{attribute 'qualified_only'}
VAR_GLOBAL
	//FFU
	FFU1_1_STATUS	:	UINT	;	//	FFU1_1运行状态
	FFU1_2_STATUS	:	UINT	;	//	FFU1_2运行状态
	FFU1_3_STATUS	:	UINT	;	//	FFU1_3运行状态
	FFU1_4_STATUS	:	UINT	;	//	FFU1_4运行状态
	FFU1_5_STATUS	:	UINT	;	//	FFU1_5运行状态
	FFU1_6_STATUS	:	UINT	;	//	FFU1_6运行状态
	FFU2_1_STATUS	:	UINT	;	//	FFU2_1运行状态
	FFU2_2_STATUS	:	UINT	;	//	FFU2_2运行状态
	FFU2_3_STATUS	:	UINT	;	//	FFU2_3运行状态
	FFU2_4_STATUS	:	UINT	;	//	FFU2_4运行状态
	FFU2_5_STATUS	:	UINT	;	//	FFU2_5运行状态
	FFU2_6_STATUS	:	UINT	;	//	FFU2_6运行状态
	FFU3_1_STATUS	:	UINT	;	//	FFU3_1运行状态
	FFU3_2_STATUS	:	UINT	;	//	FFU3_2运行状态
	FFU3_3_STATUS	:	UINT	;	//	FFU3_3运行状态
	FFU3_4_STATUS	:	UINT	;	//	FFU3_4运行状态
	FFU3_5_STATUS	:	UINT	;	//	FFU3_5运行状态
	FFU3_6_STATUS	:	UINT	;	//	FFU3_6运行状态

	FFU1_1_SPEED_PV	:	UINT	;	//	FFU1_1当前转速
	FFU1_2_SPEED_PV	:	UINT	;	//	FFU1_2当前转速
	FFU1_3_SPEED_PV	:	UINT	;	//	FFU1_3当前转速
	FFU1_4_SPEED_PV	:	UINT	;	//	FFU1_4当前转速
	FFU1_5_SPEED_PV	:	UINT	;	//	FFU1_5当前转速
	FFU1_6_SPEED_PV	:	UINT	;	//	FFU1_6当前转速
	FFU2_1_SPEED_PV	:	UINT	;	//	FFU2_1当前转速
	FFU2_2_SPEED_PV	:	UINT	;	//	FFU2_2当前转速
	FFU2_3_SPEED_PV	:	UINT	;	//	FFU2_3当前转速
	FFU2_4_SPEED_PV	:	UINT	;	//	FFU2_4当前转速
	FFU2_5_SPEED_PV	:	UINT	;	//	FFU2_5当前转速
	FFU2_6_SPEED_PV	:	UINT	;	//	FFU2_6当前转速
	FFU3_1_SPEED_PV	:	UINT	;	//	FFU3_1当前转速
	FFU3_2_SPEED_PV	:	UINT	;	//	FFU3_2当前转速
	FFU3_3_SPEED_PV	:	UINT	;	//	FFU3_3当前转速
	FFU3_4_SPEED_PV	:	UINT	;	//	FFU3_4当前转速
	FFU3_5_SPEED_PV	:	UINT	;	//	FFU3_5当前转速
	FFU3_6_SPEED_PV	:	UINT	;	//	FFU3_6当前转速


END_VAR
